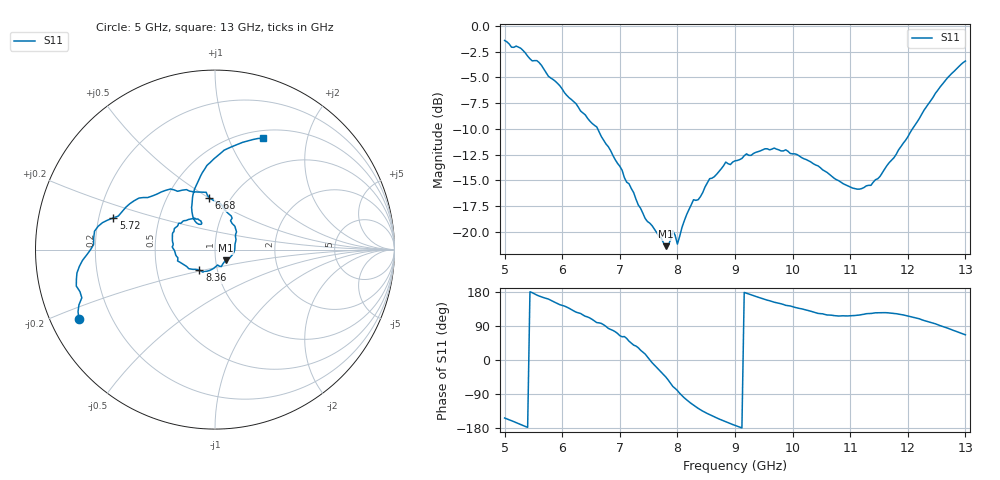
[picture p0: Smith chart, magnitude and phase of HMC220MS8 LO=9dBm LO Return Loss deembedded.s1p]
!Hittite Microwave Corporation
!12 Elizabeth Drive
!Chelmsford, MA 01824
!Tel: 978-250-3343
!Fax: 978-250-3373
!Device: HMC220MS8, 5-12 GHz, GaAS MMIC SMT Double-Balanced Mixer in 8-lead MSOP package
!Misc: LO power level=9dBm, Room
# MHZ S MA R 50
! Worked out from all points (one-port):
!   201 points, 5 GHz to 13 GHz, reference 50 ohm
!   lowest |S11| = -21.4 dB at 7.8 GHz (marker M1), VSWR 1.19, Z = 56 - j6.78 ohm
!   |S11| at or under -10 dB: 6.616 GHz to 12.08 GHz (5.465 GHz wide, 58.5 % of centre)
!   S11 on the Smith chart (normalised r, x): 5 GHz: 0.09, -0.24; 5.72 GHz: 0.26, +0.14; 6.68 GHz: 0.80, +0.50; 8.36 GHz: 0.82, -0.19; 13 GHz: 0.59, +1.35
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5000  0.851 -153.0
5280  0.78 -170.4
5480  0.677 177.6
5560  0.679 171.3
5720  0.593 162.7
6000  0.494 144.0
6240  0.419 126.3
6680  0.29 96.4
7000  0.208 64.2
7360  0.13 25.9
7800  0.085 -45.1
7920  0.101 -69.8
8000  0.087 -80.5
8280  0.143 -119.1
8360  0.143 -127.6
8560  0.181 -144.2
8840  0.218 -163.2
9000  0.221 -172.5
9520  0.253 159.7
10000  0.239 140.7
10440  0.209 123.0
11000  0.165 116.6
11360  0.168 122.7
11760  0.229 123.1
12000  0.289 116.2
12480  0.471 95.5
12760  0.587 79.8
13000  0.676 66.5
